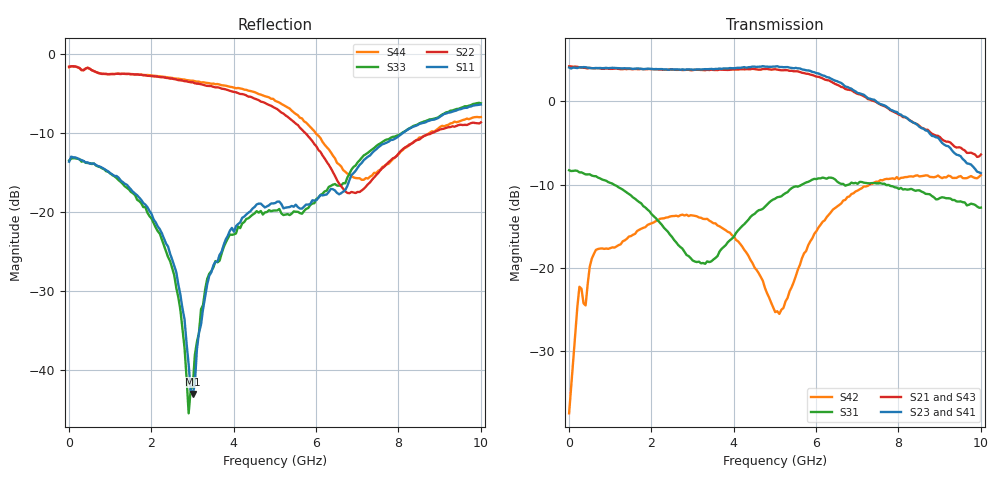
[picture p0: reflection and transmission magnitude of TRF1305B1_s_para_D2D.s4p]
! Created Thu Apr 18 17:02:45 2024
# hz S ri R 50
! 4 Port Network Data from SP1.SP block
!port1 - INP, port2 - OUTP, port3 - INM, port4 - OUTM
! freq  reS11  imS11  reS12  imS12  reS13  imS13  reS14  imS14
!  reS21  imS21  reS22  imS22  reS23  imS23  reS24  imS24
!  reS31  imS31  reS32  imS32  reS33  imS33  reS34  imS34
!  reS41  imS41  reS42  imS42  reS43  imS43  reS44  imS44
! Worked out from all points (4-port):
!   201 points, 10 MHz to 10 GHz, reference 50 ohm
!   strongest paths, dB at 10 MHz, 2.51 GHz, 5.01 GHz, 7.51 GHz, 10 GHz:
!     S23: 4.0, 3.8, 4.2, -0.2, -8.6
!     S21: 4.2, 3.8, 3.8, -0.3, -6.4
!     S41: 3.9, 3.7, 4.0, -0.1, -8.5
!     S43: 3.9, 3.7, 3.6, -0.6, -6.6
!     S31: -8.3, -16.3, -11.7, -9.9, -12.8
!     S42: -37.4, -13.8, -25.3, -9.7, -8.9
!   lowest |S11| = -43.0 dB at 3.01 GHz (marker M1), VSWR 1.01, Z = 49.4 + j0.408 ohm
!   |S11| at or under -10 dB: start of sweep to 8.113 GHz
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1e7  0.2078 -0.00451  -0.0055 -0.00132  0.3704 0.000284  -0.00204 0.0061
     1.618 -0.00586  -0.8285 -0.0163  -1.592 -0.00248  -0.0108 -0.0133
     0.3854 -0.006  -0.00428 0.0084  0.2115 0.00569  0.00552 0.00654
     -1.574 0.0303  -0.0128 0.00404  1.567 0.026  -0.8197 0.00296
3.01e9  -0.00578 0.00413  0.0313 -0.022  -0.0939 -0.0493  0.0619 -0.0179
        -0.803 -1.309  -0.3234 0.5737  0.908 1.252  0.2043 -0.0441
        -0.1023 -0.0425  0.0606 -0.0162  0.00729 0.00309  0.0322 -0.0246
        0.8945 1.23  0.2014 -0.0446  -0.814 -1.279  -0.3351 0.5865
4.71e9  0.106 0.029  -0.0106 -0.0309  0.0277 0.2185  0.038 -0.0668
        -1.498 0.4352  0.0558 0.4914  1.523 -0.558  -0.0154 -0.087
        0.0433 0.2222  0.036 -0.0698  0.0945 0.0187  -0.012 -0.0322
        1.51 -0.5043  -0.0063 -0.0835  -1.472 0.414  0.0555 0.5424
6.51e9  0.1292 0.0274  0.00556 -0.00587  0.3271 0.0944  -0.0254 -0.0875
        0.3995 1.191  0.0708 0.1422  -0.4647 -1.234  0.0686 0.2349
        0.3221 0.0727  -0.0279 -0.0847  0.1421 0.0372  0.00527 -0.00893
        -0.3988 -1.271  0.0646 0.224  0.3813 1.156  0.1029 0.1764
6.71e9  0.1277 0.0507  2.49e-05 -4.08e-05  0.3155 0.0716  -0.0399 -0.0751
        0.5495 1.048  0.0338 0.1307  -0.608 -1.063  0.0992 0.2452
        0.3053 0.0626  -0.0416 -0.0717  0.1428 0.0519  -0.0014 -0.00479
        -0.5679 -1.109  0.1003 0.2355  0.5293 1.016  0.0709 0.1651
7.01e9  0.1765 0.0717  0.0108 0.00749  0.3336 0.0439  -0.0433 -0.0614
        0.7424 0.82  -0.00982 0.1336  -0.7682 -0.816  0.1671 0.2488
        0.3181 0.0318  -0.0425 -0.0563  0.1964 0.062  0.0064 0.0024
        -0.7512 -0.8598  0.1689 0.2372  0.6987 0.7958  0.0253 0.1614
1e10  0.3097 -0.3635  0.0119 -0.096  0.0914 -0.2231  -0.0522 -0.0465
      0.1521 -0.4536  0.0326 0.3668  -0.1909 0.3175  0.3838 -0.1076
      0.0923 -0.2108  -0.0459 -0.0574  0.252 -0.416  0.00011 -0.0879
      -0.2123 0.3116  0.3455 -0.1038  0.1515 -0.4423  -0.00529 0.3977
